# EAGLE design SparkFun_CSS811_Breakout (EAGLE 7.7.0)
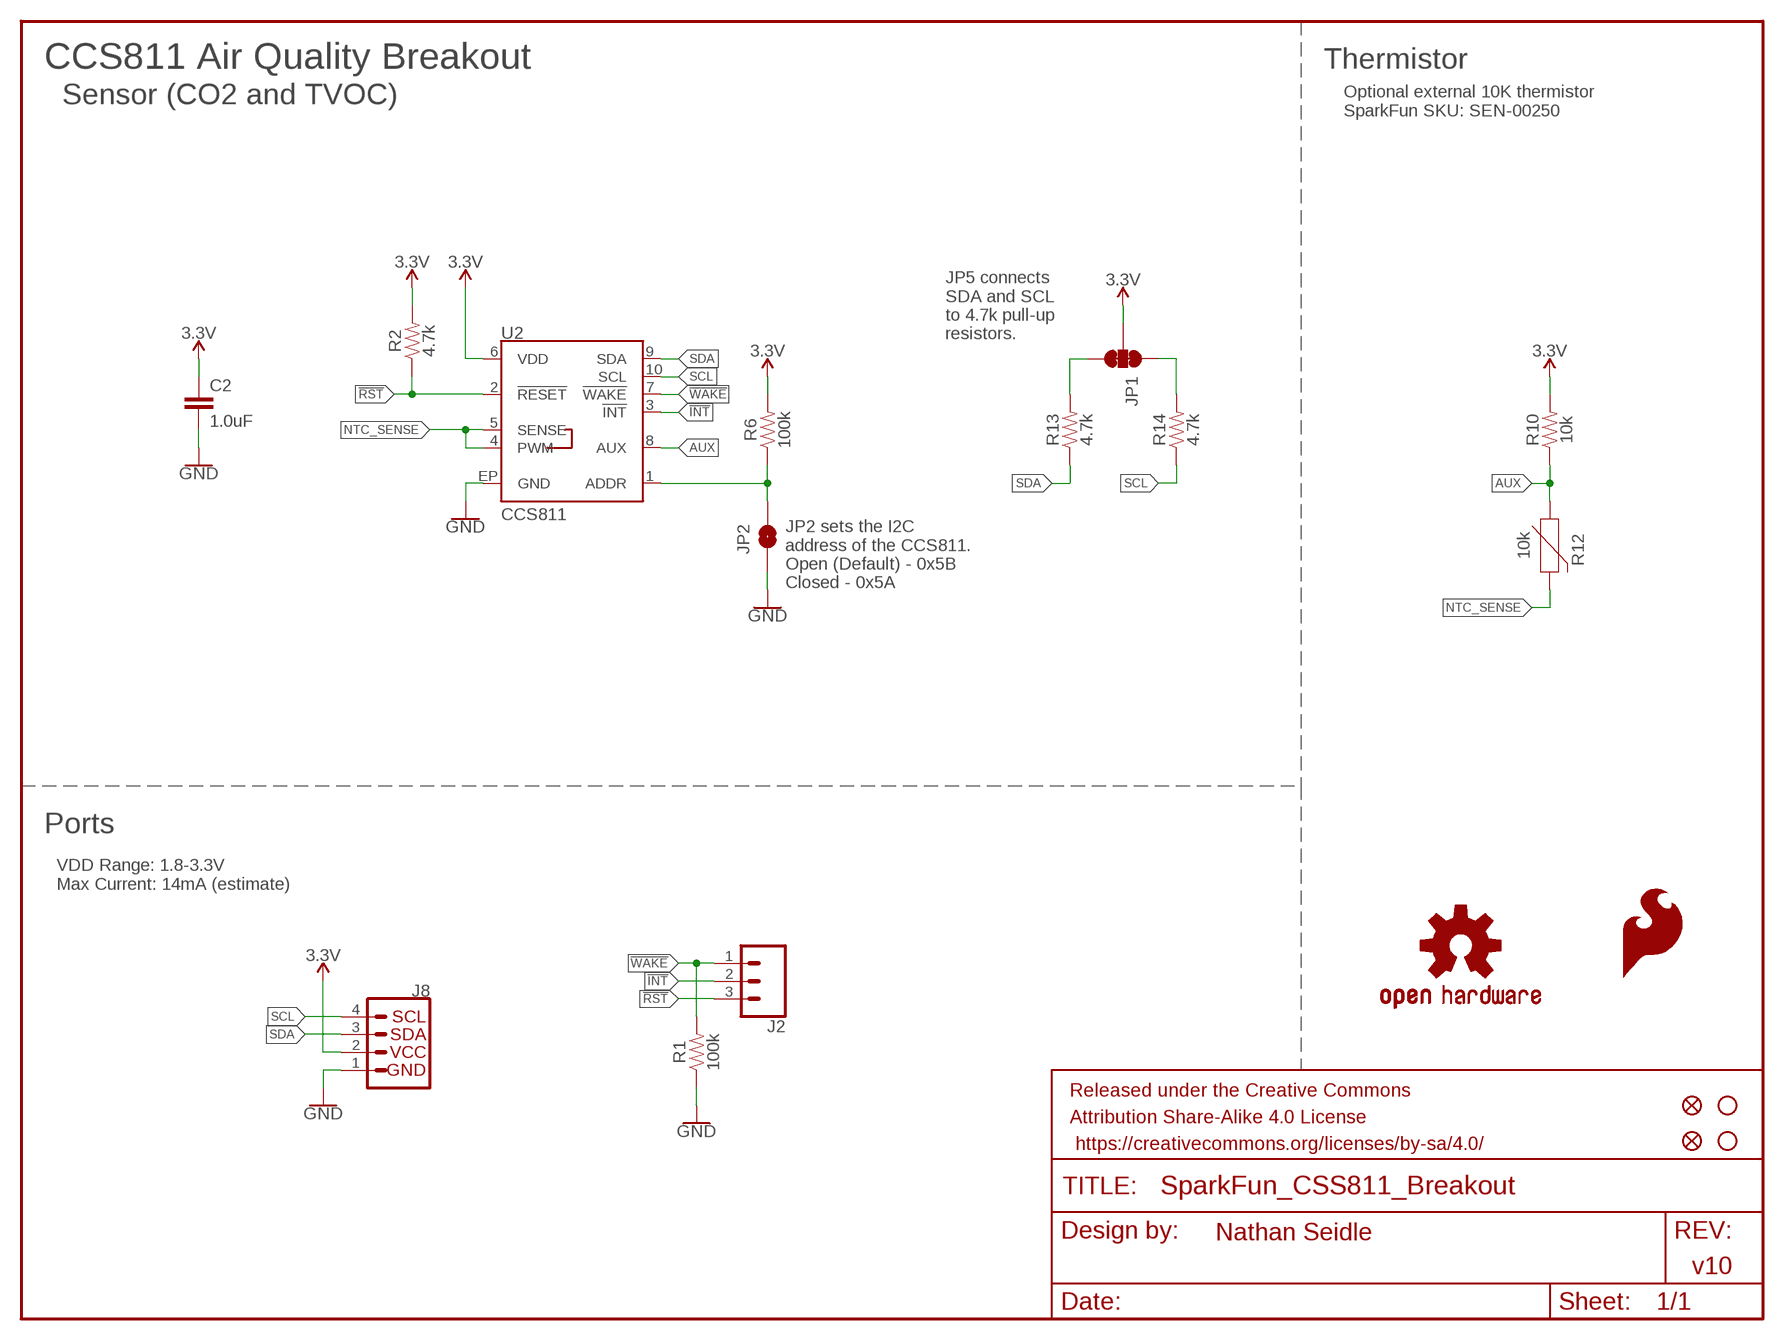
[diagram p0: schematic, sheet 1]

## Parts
C2  1.0uF  1.0UF-0603-16V-10%  [0603]
FD1  FIDUCIAL1X2  [FIDUCIAL-1X2]
FD2  FIDUCIAL1X2  [FIDUCIAL-1X2]
FRAME1  FRAME-LETTER  [CREATIVE_COMMONS]
H2  STAND-OFF  [STAND-OFF]
H4  STAND-OFF  [STAND-OFF]
J2  CONN_031X03_NO_SILK  [1X03_NO_SILK]
J8  I2C_STANDARD_NO_SILK  [1X04_NO_SILK]
JP1  JUMPER-SMT_3_2-NC_TRACE_SILK  [SMT-JUMPER_3_2-NC_TRACE_SILK]
JP2  JUMPER-SMT_2_NO_SILK  [SMT-JUMPER_2_NO_SILK]
LOGO1  SFE_LOGO_FLAME.2_INCH  [SFE_LOGO_FLAME_.2]
LOGO4  OSHW-LOGOS  [OSHW-LOGO-S]
R1  100k  100KOHM-0603-1/10W-1%  [0603]
R2  4.7k  4.7KOHM-0603-1/10W-1%  [0603]
R6  100k  100KOHM-0603-1/10W-1%  [0603]
R10  10k  10KOHM-0603-1/10W-1%  [0603]
R12  10k  NTC-THERMISTOR-AXIAL-0.1  [AXIAL-0.1]
R13  4.7k  4.7KOHM-0603-1/10W-1%  [0603]
R14  4.7k  4.7KOHM-0603-1/10W-1%  [0603]
U2  CCS811  [LGA10]

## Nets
3.3V: C2.1 J8.2 JP1.2 R2.2 R6.2 R10.2 U2.6(VDD)
!INT: J2.2 U2.3(!INT!)
!RST: J2.3 R2.1 U2.2(!RESET!)
!WAKE: J2.1 R1.2 U2.7(!WAKE!)
AUX: R10.1 R12.P$1 U2.8(AUX)
CCS811_ADDR: JP2.2 R6.1 U2.1(ADDR)
GND: C2.2 J8.1 JP2.1 R1.1 U2.EP(GND)
N$4: JP1.3 R13.2
N$5: JP1.1 R14.2
NTC_SENSE: R12.P$2 U2.4(PWM) U2.5(SENSE)
SCL: J8.4 R14.1 U2.10(SCL)
SDA: J8.3 R13.1 U2.9(SDA)

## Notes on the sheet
- CCS811 Air Quality Breakout | Thermistor
- Optional external 10K thermistor
  SparkFun SKU: SEN-00250
- Sensor (CO2 and TVOC)
- JP5 connects 
  SDA and SCL 
  to 4.7k pull-up 
  resistors.
- JP2 sets the I2C 
  address of the CCS811.
  Open (Default) - 0x5B
  Closed - 0x5A
- Ports
- VDD Range: 1.8-3.3V
  Max Current: 14mA (estimate)
- Nathan Seidle
- v10

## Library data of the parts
C2 = SparkFun-Capacitors:1.0UF: 1µF ceramic capacitors; PROD_ID: CAP-00868
FD1 FD2 = SparkFun-Aesthetics:FIDUCIAL: Fiducial Alignment Points
FRAME1 = SparkFun-Aesthetics:FRAME-LETTER: Schematic Frame - Letter
H2 H4 = SparkFun-Hardware:STAND-OFF: Stand Off
J2 = SparkFun-Connectors:CONN_03: Multi connection point. Often used as Generic Header-pin footprint for 0.1 inch spaced/style header connections On any of the 0.1 inch spaced packages, you can populate with these: Break Away Headers - Straight (PRT-00116) Break Away Male Headers - Right Angle (PRT-00553) Female Headers (PRT-00115)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
J8 = SparkFun-Connectors:I2C_STANDARD: SparkFun I2C Standard Pinout Header SparkFun has standardized on a pinout for all I2C based sensor breakouts. This pinout allows I2C boards to be plugged directly into the headers on Arduino Uno compatible boards, and to be daisy chained easily. Example SparkFun Products: SparkFun Atmospheric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
JP1 = SparkFun-Jumpers:JUMPER-SMT_3_2-NC_TRACE: Normally closed trace jumper (2 of 2 connections) This jumper has a trace between all three pads so they are normally closed (NC). Use a razor knife to open the connection(s). For best results follow the IPC guidelines for cutting traces: Cutout at least 0.063 mm (0.005 in). Remove all loose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
JP2 = SparkFun-Jumpers:JUMPER-SMT_2_NO: Normally open jumper
LOGO1 = SparkFun-Aesthetics:SFE_LOGO_FLAME: SparkFun Flame Logo
LOGO4 = SparkFun-Aesthetics:OSHW-LOGO: Open-Source Hardware (OSHW) Logo
R1 R6 = SparkFun-Resistors:100KOHM: 100kΩ resistor; PROD_ID: RES-07828
R2 R13 R14 = SparkFun-Resistors:4.7KOHM: 4.7kΩ resistor; PROD_ID: RES-07857
R10 = SparkFun-Resistors:10KOHM: 10kΩ resistor; PROD_ID: RES-00824
R12 = CCS811_Breakout_Temp:NTC-THERMISTOR: NTC Thermistor; PROD_ID: N/A; SF_ID: SEN-00250
U2 = CCS811_Breakout_Temp:CCS811: AMS CCS811 &ndash; I2C Digital Gas Sensor Ultra-Low Power Digital Gas Sensor for Monitoring Indoor Air Quality AMS Product Page SparkFun Products:; PROD_ID: IC-13607

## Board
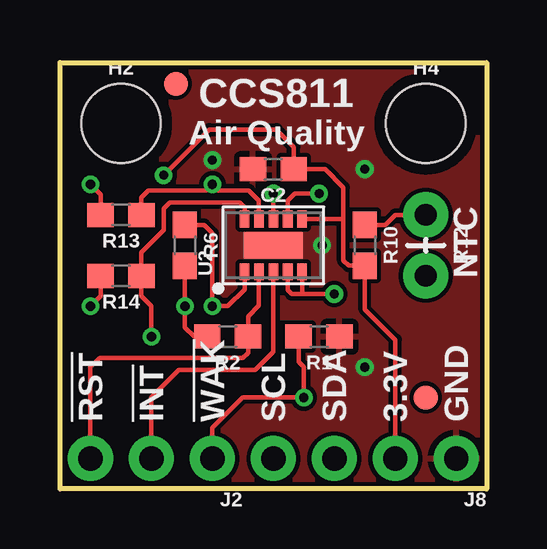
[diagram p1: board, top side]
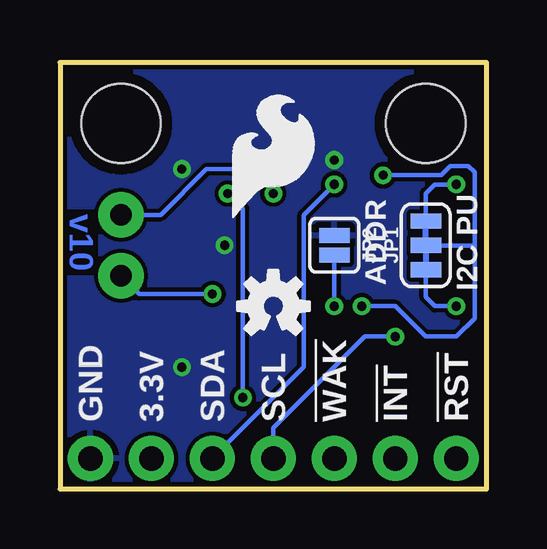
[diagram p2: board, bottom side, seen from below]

Size 17.78 x 17.78 mm. Coordinates in mm from the lower left corner, seen from the top.
Outline: 0,0 0,17.78 17.78,17.78 17.78,0 0,0
Copper layers (1*16): Top 0.035mm / dielectric 1.5mm / Bottom 0.035mm
Design rules "SparkFun-2-layer-TIGHT": minimum track width 7mil, minimum drill 15mil, track to track 7mil, track to pad 7mil, pad to pad 7mil, via to via 7mil, smd to smd 7mil, copper to edge 7mil, drill to drill 7mil, minimum pad ring 7mil, minimum via ring 7mil, stop-mask expansion 4mil, vias tented up to drill 25mil, thermal gap 10mil

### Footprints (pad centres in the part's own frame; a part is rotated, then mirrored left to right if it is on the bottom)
0603 = smd 1.1 x 1: 1 -0.85,0; 2 0.85,0
FIDUCIAL-1X2 = smd 1 x 1: 1 0,0
STAND-OFF = hole 3.302: 0,0
1X03_NO_SILK = drill 1.016 pad 1.88: 1 0,0; 2 2.54,0; 3 5.08,0
1X04_NO_SILK = drill 1.016 pad 1.88: 1 0,0; 2 2.54,0; 3 5.08,0; 4 7.62,0
SMT-JUMPER_3_2-NC_TRACE_SILK = smd 0.635 x 1.27: 1 -1.016,0; 2 0,0; 3 1.016,0
SMT-JUMPER_2_NO_SILK = smd 0.635 x 1.27: 1 -0.406,0; 2 0.406,0
AXIAL-0.1 = drill 0.9 pad 1.88: P$1 -1.27,0; P$2 1.27,0
LGA10 = smd 0.7 x 0.4: 1 -1.1,1.2; 2 -1.1,0.6; 3 -1.1,0; 4 -1.1,-0.6; 5 -1.1,-1.2; 6 1.1,-1.2; 7 1.1,-0.6; 8 1.1,0; 9 1.1,0.6; 10 1.1,1.2 | smd 1.1 x 2.45: EP 0,0

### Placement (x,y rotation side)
C2  8.89,13.34 180 top
FD1  4.83,16.89 0 top
FD2  15.24,3.81 0 top
FRAME1  not placed on the board
H2  2.54,15.24 0 top
H4  15.24,15.24 0 top
J2  6.35,1.27 180 top
J8  16.51,1.27 180 top
JP1  2.54,10.16 90 bottom
JP2  6.35,10.16 270 bottom
LOGO1  10.92,11.05 0 bottom
LOGO4  8.89,7.62 0 bottom
R1  10.79,6.35 180 top
R2  6.99,6.35 180 top
R6  5.21,10.16 270 top
R10  12.7,10.16 270 top
R12  15.24,10.16 270 top
R13  2.54,11.43 180 top
R14  2.54,8.89 180 top
U2  8.89,10.16 90 top

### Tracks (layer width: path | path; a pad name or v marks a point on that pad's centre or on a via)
3.3V  (via drill 0.38)
  Top 0.178: J8.2 13.97,6.22 12.7,7.49 R10.2 12.03,9.31 11.81,9.53 11.81,11.3 | U2.6 11.77,11.26 11.81,11.3 | v4.32,13.08 6.22,14.99 9.02,14.99 9.74,14.26 C2.1 11.05,13.34 11.81,12.57 11.81,11.3 | R6.2 v5.21,7.62 5.21,6.73 5.59,6.35 R2.2
  Bottom 0.178: v4.32,13.08 1.91,13.08 1.52,13.46 0.76,13.46 0.51,13.21 0.51,10.16 | 0.51,10.16 0.51,7.11 1.27,6.35 2.54,6.35 3.81,7.62 v5.21,7.62 | JP1.2 0.51,10.16
!INT
  Top 0.178: U2.3 8.89,5.71 8.13,4.95 4.95,4.95 3.81,3.81 J2.2
!RST
  Top 0.178: U2.2 8.29,7.66 7.83,7.2 R2.1 7.83,5.68 7.62,5.46 1.65,5.46 1.27,5.08 J2.3
!WAKE  (via drill 0.38)
  Top 0.178: U2.7 9.49,12.03 9.78,12.32 v10.79,12.32 | J2.1 6.35,2.54 7.62,3.81 v10.16,3.81 10.16,5.08 9.95,5.29 R1.2
  Bottom 0.178: v10.16,3.81 10.16,11.68 v10.79,12.32
AUX  (via drill 0.38)
  Top 0.178: R10.1 13.55,11.01 13.97,11.43 R12.P$1 | U2.8 v8.89,12.32
  Bottom 0.178: v8.89,12.32 8.89,12.95 9.27,13.34 11.68,13.34 13.59,11.43 R12.P$1
CCS811_ADDR  (via drill 0.38)
  Top 0.178: R6.1 6.01,11.01 6.35,10.67 v6.35,7.62 6.99,7.62 7.69,8.32 U2.1
  Bottom 0.178: JP2.2 v6.35,7.62
GND  (via drill 0.38)
  other vias: 6.35,13.72 10.92,10.16 12.7,13.34 12.7,5.08
  pour Top (isolate 0.178): 0,0 17.78,0 17.78,17.78 0,17.78
  pour Bottom (isolate 0.178): 0,17.78 17.78,17.78 17.78,0 0,0
N$4  (via drill 0.38)
  Top 0.178: R13.2 1.69,12.28 v1.27,12.7
  Bottom 0.178: v1.27,12.7 2.16,12.7 2.54,12.32 JP1.3
N$5  (via drill 0.38)
  Top 0.178: R14.2 1.69,8.04 v1.27,7.62
  Bottom 0.178: v1.27,7.62 2.16,7.62 2.54,8 JP1.1
NTC_SENSE  (via drill 0.38)
  Top 0.178: 10.16,8.13 9.65,8.13 9.49,8.29 U2.4 | 10.16,8.13 v11.43,8.13 | U2.5 10.09,8.2 10.16,8.13
  Bottom 0.178: v11.43,8.13 14.48,8.13 R12.P$2
SCL  (via drill 0.38)
  Top 0.178: v3.81,6.35 3.81,7.62 3.39,8.04 R14.1 3.39,9.87 4.32,10.79 4.32,11.68 4.57,11.94 7.49,11.94 7.69,11.74 U2.10
  Bottom 0.178: v3.81,6.35 5.08,6.35 8.89,2.54 J8.4
SDA  (via drill 0.38)
  Top 0.178: R13.1 3.39,12.15 3.68,12.45 6.1,12.45 v6.35,12.7 6.6,12.45 7.87,12.45 8.29,12.03 U2.9
  Bottom 0.178: J8.3 7.62,5.08 7.62,11.43 v6.35,12.7

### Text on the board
Bottom: v10
tPlace: CCS811 | Air Quality | NTC | !RST | !INT | !WAK | SCL | SDA | 3.3V | GND
bPlace: I2C PU | ADDR | !RST | !INT | !WAK | SCL | SDA | 3.3V | GND
Measures: All measurements in inches
tDocu: Nathan Seidle

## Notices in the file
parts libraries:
SparkFun-Aesthetics: Licensing: Creative Commons ShareAlike 4.0 International - https://creativecommons.org/licenses/by-sa/4.0
SparkFun-Aesthetics: Released under the Creative Commons Attribution Share-Alike 4.0 License
SparkFun-Aesthetics: https://creativecommons.org/licenses/by-sa/4.0
